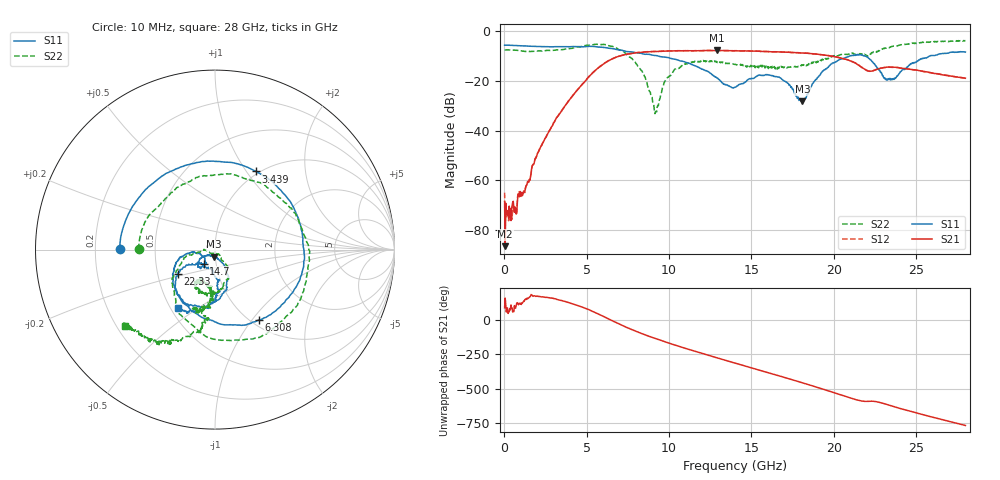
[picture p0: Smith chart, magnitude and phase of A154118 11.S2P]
!  2-Port S-parameters saved by WinCal
! VAR MeasName=S-Parameters (CALIBRATED_DATA) read from VNA (N5230A)
! VAR MeasDate=2015-9-10 14:35:13
! VAR NAME=A154118 11
! VAR FILENAME=A154118 11.S2P
! VAR DATE=2015-9-10 14:35:13
! VAR PHYS_PORTS=1,2
# Hz S DB R 50
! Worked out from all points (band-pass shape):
!   801 points, 10 MHz to 28 GHz, reference 50 ohm
!   highest |S21| = -7.63 dB at 12.89 GHz (marker M1); lowest = -86.5 dB at 44.99 MHz (marker M2)
!   |S21| within 3 dB of the highest: 6.677 GHz to 20.37 GHz (13.7 GHz wide, 101 % of centre)
!   lowest |S11| = -28.1 dB at 18.1 GHz (marker M3), VSWR 1.08, Z = 49.4 - j3.87 ohm
!   |S11| at or under -10 dB: 9.398 GHz to 20.93 GHz (11.53 GHz wide, 76 % of centre); 21.90578 GHz to 21.93241 GHz (26.64 MHz wide, 0.122 % of centre); 21.96 GHz to 25.79 GHz (3.833 GHz wide, 16.1 % of centre)
!   |S22| runs from -33.1 to -3.6 dB; largest |S21 - S12| = 0.007
!   S11 on the Smith chart (normalised r, x): 10 MHz: 0.31, +0.00; 3.439 GHz: 0.97, +1.11; 6.308 GHz: 1.09, -1.08; 14.7 GHz: 0.87, -0.14; 22.33 GHz: 0.64, -0.18; 28 GHz: 0.54, -0.41
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1e7  -5.54 179.5  -68.47 89.3  -64.95 49.1  -7.50 179.8
4.49875e7  -5.52 178.5  -86.49 159.8  -78.88 -114.8  -7.46 178.7
6.047875e8  -5.64 160.1  -72.84 104.8  -72.52 84.9  -7.53 161.5
3.438775e9  -6.17 62.3  -32.32 142.7  -32.28 142.5  -7.36 71.3
4.698325e9  -6.14 8.3  -21.50 95.0  -21.46 94.9  -6.04 12.9
6.30775e9  -6.73 -58.1  -11.82 9.3  -11.79 9.1  -5.65 -74.8
7.602288e9  -8.17 -96.5  -8.99 -62.8  -8.95 -62.9  -10.32 -141.1
8.441988e9  -9.08 -114.9  -8.32 -103.0  -8.26 -103.2  -16.79 -168.4
9.141738e9  -9.68 -128.4  -8.08 -133.6  -8.03 -134.1  -33.11 -115.5
9.351662e9  -9.90 -132.2  -8.06 -142.2  -8.00 -142.6  -29.88 -52.8
9.736525e9  -10.32 -137.8  -7.90 -157.6  -7.87 -158.0  -20.23 -52.8
1.040129e10  -11.25 -149.7  -7.79 176.3  -7.78 175.6  -15.06 -65.9
1.28854e10  -18.60 -172.9  -7.63 86.2  -7.63 85.6  -12.02 -111.6
1.4005e10  -22.51 -140.1  -7.78 46.9  -7.77 46.5  -13.25 -121.0
1.470475e10  -19.94 -128.4  -7.84 22.4  -7.81 21.9  -14.35 -118.2
1.662906e10  -18.40 -143.1  -8.20 -44.0  -8.18 -44.6  -14.78 -112.8
1.809854e10  -28.07 -97.2  -8.70 -96.2  -8.74 -96.8  -13.59 -98.5
1.869332e10  -21.16 -60.9  -8.94 -118.1  -9.00 -118.3  -12.32 -93.7
2.040771e10  -11.21 -84.7  -10.72 176.8  -10.67 176.4  -9.32 -100.6
2.233202e10  -12.15 -147.1  -15.92 129.4  -15.93 128.7  -8.57 -98.1
2.334666e10  -19.39 -120.3  -14.34 101.5  -14.35 100.9  -6.53 -102.9
2.8e10  -8.29 -122.6  -18.82 -46.6  -18.85 -47.0  -3.62 -139.8
